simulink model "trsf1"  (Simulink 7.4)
settings: Solver=ode23  StartTime=0.0  StopTime=1  MaxStep=0.5e-3  RelTol=1e-3  AbsTol=1e-3
libraries: simulink x1

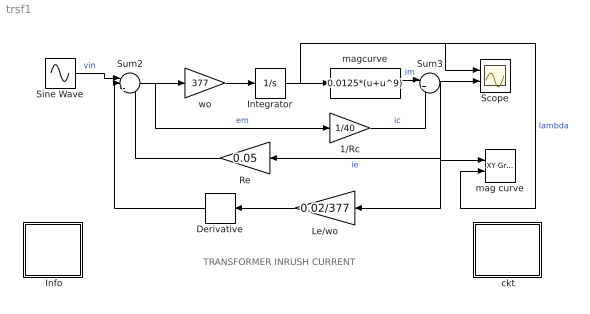
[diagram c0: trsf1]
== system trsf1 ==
  note: TRANSFORMER INRUSH CURRENT
  " Info" : Subsystem
  " ckt" : Subsystem
  1/Rc : Gain  Gain=1/40  ParameterDataType=sfix(16)  ParameterScaling=2^0  OutDataType=sfix(16)  OutScaling=2^0
  Derivative : Derivative
  Integrator : Integrator
  Le/wo : Gain  Gain=0.02/377  ParameterDataType=sfix(16)  ParameterScaling=2^0  OutDataType=sfix(16)  OutScaling=2^0
  Re : Gain  Gain=0.05  ParameterDataType=sfix(16)  ParameterScaling=2^0  OutDataType=sfix(16)  OutScaling=2^0
  Scope : Scope  NumInputPorts=2
  Sine Wave : Sin  Amplitude=1.0  Bias=0  Frequency=2*pi*50  Phase=0  Samples=10  SampleTime=0
  Sum2 : Sum  Inputs=|+--  OutDataType=sfix(16)  OutScaling=2^0
  Sum3 : Sum  Inputs=|++  OutDataType=sfix(16)  OutScaling=2^0
  mag curve : simulink/Sinks/XY Graph  SystemSampleTime=-1  xmin=-2  xmax=2  ymin=-2  ymax=2  st=-1
  magcurve : Fcn  Expr=0.0125*(u+u^9)
  wo : Gain  Gain=377  ParameterDataType=sfix(16)  ParameterScaling=2^0  OutDataType=sfix(16)  OutScaling=2^0
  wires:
  wo/1 -> Integrator/1
  Re/1 -> Sum2/3
  Sine Wave/1 -> Sum2/1  "vin"
  Integrator/1 -> magcurve/1, Scope/1, mag curve/2  "lambda"
  Sum2/1 -> wo/1, 1/Rc/1  "em"
  1/Rc/1 -> Sum3/2  "ic"
  magcurve/1 -> Sum3/1  "im"
  Sum3/1 -> Scope/2, mag curve/1, Le/wo/1, Re/1  "ie"
  Derivative/1 -> Sum2/2
  Le/wo/1 -> Derivative/1

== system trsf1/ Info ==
  note: This demo simulates the inrush current phenomenon following the application of a sinusoidal voltage source to a transformer under open circuit. (per-unit system representation) The instant of closure is adjusted by specifying the phase angle of the sinusoidal source.

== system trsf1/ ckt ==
  note: This demo simulates the running of an induction motor in steady-state when a sudden input change is effected: a)torque step changes at constant voltage excitation b) voltage input sag at constant frequency and load torque c)simultaneous step changes in voltage magnitude and frequency
  note: Double click the block to enter the machine parameters and initial conditions and then run the simulation
